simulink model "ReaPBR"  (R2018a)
settings: Solver=VariableStepAuto  StartTime=0.0  StopTime=10000  RelTol=1e-3
undefined symbols (not defined in the file): a7dd, ac9bf013aa13, b045, c0379df8, d9caee96080d, ReaPBR, sdiscope

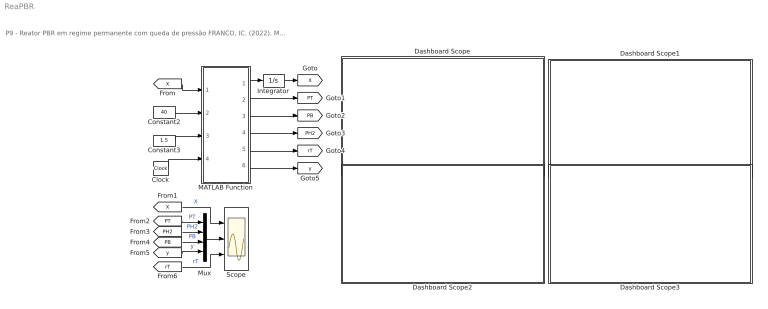
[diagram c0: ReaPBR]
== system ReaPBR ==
  note: P9 - Reator PBR em regime permanente com queda de pressão FRANCO, IC. (2022). Modelagem e Simulação: Problemas Típicos da Engenharia Química para Simulação e Análise. NOTAS DE AULA INOVADORAS. The Journal of Engineering and Exact Sciences. Material Complementar.
  Clock : Clock
  Constant2 : Constant  Value=40
  Constant3 : Constant  Value=1.5
  Dashboard Scope : Subsystem  DialogController=hmiCreateDDGDialog  IsWebBlock=on  mask(MWDashboardBlock){webBlockId=6482c64e-62b0-475b-8caa-3c66be80ba74, webBlockType=sdiscope, ShowInitialText=on, HMISrcModelName=ReaPBR}
      mask prompts: webBlockId "WebBlock Id"; webBlockType "WebBlock Type"; HMISrcModelName "Source Model"
      mask help: SimulinkHMI:dialogs:HMIScopeDialogDesc
  Dashboard Scope1 : Subsystem  DialogController=hmiCreateDDGDialog  IsWebBlock=on  mask(MWDashboardBlock){webBlockId=c0379df8-27ab-4ba9-a7dd-d9caee96080d, webBlockType=sdiscope, ShowInitialText=on, HMISrcModelName=ReaPBR}
      mask prompts: webBlockId "WebBlock Id"; webBlockType "WebBlock Type"; HMISrcModelName "Source Model"
      mask help: SimulinkHMI:dialogs:HMIScopeDialogDesc
  Dashboard Scope2 : Subsystem  DialogController=hmiCreateDDGDialog  IsWebBlock=on  mask(MWDashboardBlock){webBlockId=03cb1a51-8177-45f3-b045-ac9bf013aa13, webBlockType=sdiscope, ShowInitialText=on, HMISrcModelName=ReaPBR}
      mask prompts: webBlockId "WebBlock Id"; webBlockType "WebBlock Type"; HMISrcModelName "Source Model"
      mask help: SimulinkHMI:dialogs:HMIScopeDialogDesc
  Dashboard Scope3 : Subsystem  DialogController=hmiCreateDDGDialog  IsWebBlock=on  mask(MWDashboardBlock){webBlockId=8464fe47-59a3-47c5-9658-99cf7b803921, webBlockType=sdiscope, ShowInitialText=on, HMISrcModelName=ReaPBR}
      mask prompts: webBlockId "WebBlock Id"; webBlockType "WebBlock Type"; HMISrcModelName "Source Model"
      mask help: SimulinkHMI:dialogs:HMIScopeDialogDesc
  Integrator : Integrator
  MATLAB Function : MATLAB Function  TreatAsAtomicUnit=on
  Mux : Mux
  Scope : Scope  NumInputPorts=3
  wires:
  Integrator/1 -> [X]
  [X] -> MATLAB Function/1(X)
  MATLAB Function/1(dX) -> Integrator/1
  MATLAB Function/2(PT) -> [PT]
  MATLAB Function/3(PB) -> [PB]
  MATLAB Function/4(PH2) -> [PH2]
  MATLAB Function/5(rT) -> [rT]
  MATLAB Function/6(y) -> [y]
  Constant2/1 -> MATLAB Function/2(P0)
  Constant3/1 -> MATLAB Function/3(Theta)
  Clock/1 -> MATLAB Function/4(W)
  [X] -> Scope/1  "X"
  [PT] -> Mux/1  "PT"
  [PH2] -> Mux/2  "PH2"
  [PB] -> Mux/3  "PB"
  [y] -> Mux/4  "y"
  [rT] -> Scope/3  "rT"
  Mux/1 -> Scope/2

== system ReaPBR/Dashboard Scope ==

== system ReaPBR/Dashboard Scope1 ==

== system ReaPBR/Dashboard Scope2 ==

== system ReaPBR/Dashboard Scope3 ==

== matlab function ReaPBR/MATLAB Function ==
function [dX,PT,PB,PH2,rT,y] = fcn(X,P0,Theta,W)
%% Parâmetros
FT0   = 5.000e+1;
k     = 8.700e-4;
KB    = 1.390;
KT    = 1.038;
alpha = 9.800e-5;

%% Equações auxiliares;
y  = (1-alpha*W)^0.5;
PT0= 0.3*P0;
PT = PT0*(1-X)*y;
PH2= PT0*(Theta-X)*y;
PB = PT0*X*y;
rT = -k*PH2*PT/(1+KB*PB+KT*PT);

%% Modelo matemático
dX = -rT/FT0;
end
